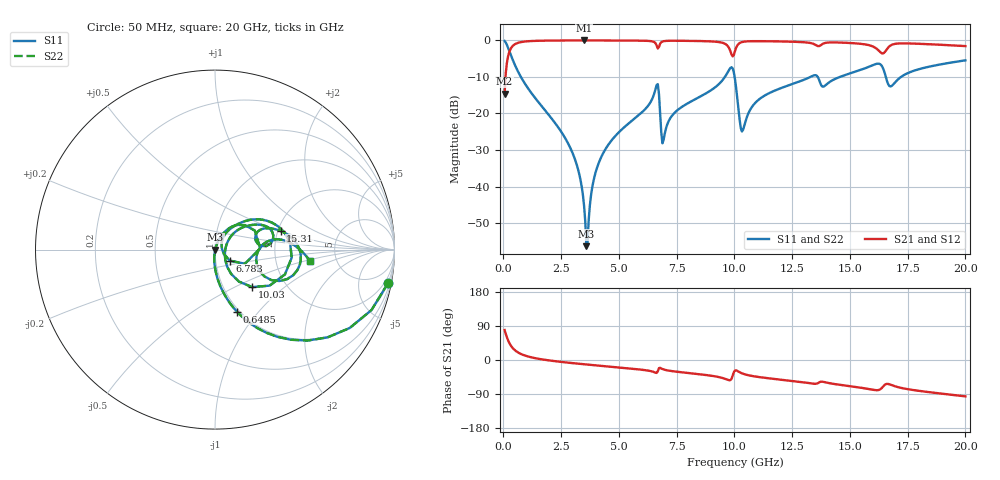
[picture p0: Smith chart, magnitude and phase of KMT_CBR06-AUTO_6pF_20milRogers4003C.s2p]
! Data measured by Modelithics Inc. support@modelithics.com 813-866-6335
! KEMET CBR06-AUTO 6pF, Pad Width= 0.851mm, Pad Length= 0.64mm, Pad Gap= 0.62mm, 20mil Rogers 4003C substrate Data, January 2022
# hz S ma R 50
! 2 Port Network Data from SP1.SP block
! freq  magS11  angS11  magS21  angS21  magS12  angS12  magS22  angS22
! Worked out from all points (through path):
!   401 points, 50 MHz to 20 GHz, reference 50 ohm
!   highest |S21| = -0.01 dB at 3.491 GHz (marker M1); lowest = -14.6 dB at 50 MHz (marker M2)
!   group delay of S21, straight-line fit = 14.8 ps
!   lowest |S11| = -56.3 dB at 3.591 GHz (marker M3), VSWR 1.00, Z = 50.1 - j0.12 ohm
!   |S11| at or under -10 dB: 755.9 MHz to 9.587 GHz (8.831 GHz wide, 171 % of centre); 10.01 GHz to 13.29 GHz (3.278 GHz wide, 28.1 % of centre); 13.61 GHz to 14.56 GHz (956 MHz wide, 6.79 % of centre)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
!   |S22| runs from -56.3 to -0.2 dB; largest |S21 - S12| = 0
!   S11 on the Smith chart (normalised r, x): 50 MHz: 1, -10; 648.5 MHz: 0.97, -0.77; 6.783 GHz: 1.17, -0.14; 10.03 GHz: 1.36, -0.62; 15.31 GHz: 2.07, +0.50; 20 GHz: 3.18, -0.57
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5e7  0.9823 -10.9  0.1868 79.1  0.1868 79.1  0.9823 -10.9
2.495e8  0.7236 -44.4  0.6897 45.5  0.6897 45.5  0.7236 -44.4
6.485e8  0.3657 -70.6  0.9301 19.3  0.9301 19.3  0.3657 -70.6
2.74325e9  0.04199 -95.3  0.998 -6.7  0.998 -6.7  0.04199 -95.3
3.391625e9  0.00982 -94.0  0.9987 -10.7  0.9987 -10.7  0.00982 -94.0
3.491375e9  0.005441 -89.0  0.9987 -11.2  0.9987 -11.2  0.005441 -89.0
3.591125e9  0.001528 -51.6  0.9987 -11.8  0.9987 -11.8  0.001528 -51.6
3.94025e9  0.01365 71.0  0.9985 -13.8  0.9985 -13.8  0.01365 71.0
4.389125e9  0.03146 71.2  0.998 -16.3  0.998 -16.3  0.03146 71.2
6.583625e9  0.2151 39.3  0.9148 -33.5  0.9148 -33.5  0.2151 39.3
6.73325e9  0.1844 -25.3  0.8157 -21.5  0.8157 -21.5  0.1844 -25.3
6.783125e9  0.1025 -36.7  0.9008 -20.7  0.9008 -20.7  0.1025 -36.7
6.93275e9  0.04345 32.7  0.9758 -24.9  0.9758 -24.9  0.04345 32.7
9.52625e9  0.297 34.6  0.9186 -48.3  0.9186 -48.3  0.297 34.6
1.0025e10  0.2943 -45.2  0.7151 -27.7  0.7151 -27.7  0.2943 -45.2
1.037412e10  0.05979 9.1  0.9568 -36.3  0.9568 -36.3  0.05979 9.1
1.112225e10  0.1609 41.0  0.9768 -45.5  0.9768 -45.5  0.1609 41.0
1.336662e10  0.325 21.4  0.9094 -62.2  0.9094 -62.2  0.325 21.4
1.531175e10  0.38 15.8  0.9082 -71.7  0.9082 -71.7  0.38 15.8
1.625938e10  0.4801 -10.1  0.7203 -78.9  0.7203 -78.9  0.4801 -10.1
1.670825e10  0.2376 -14.6  0.8285 -64.1  0.8285 -64.1  0.2376 -14.6
2e10  0.5339 -6.9  0.8358 -96.0  0.8358 -96.0  0.5339 -6.9
